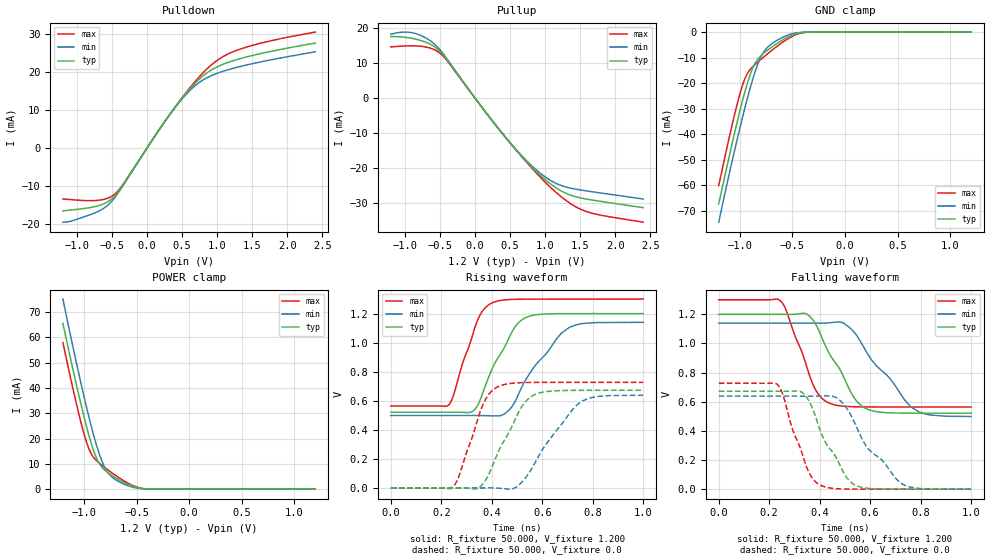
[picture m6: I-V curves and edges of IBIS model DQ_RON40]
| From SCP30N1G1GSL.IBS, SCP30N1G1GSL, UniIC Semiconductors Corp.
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|   Model DQ_RON40
[Model] DQ_RON40
Model_type I/O
Vinl =  0.500V
Vinh =  0.700V
Vmeas =  0.600V
Rref =  50.000
Vref =  0.600V
C_comp   1.373pF   1.353pF   1.403pF
[Model Spec]
Vinh   0.700V   0.670V   0.750V
Vinl   0.500V   0.470V   0.550V
Vmeas   0.600V   0.570V   0.650V
Vref   0.600V   0.570V   0.650V
Rref   50.000   NA   NA
[Temperature Range]   25.000   85.000   -40.000
[Voltage Range]   1.200V   1.140V   1.300V
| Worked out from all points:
|   slope of the pulldown table from 0 to 0.18 V, typ, clamps not added: 36 ohm
|   slope of the pullup table from 0 to 0.18 V, typ, clamps not added: 37.6 ohm
|   GND clamp passes 1 mA (typ) near -0.49 V on its own axis
|   POWER clamp passes 1 mA (typ) near -0.53 V on its own axis
|   rising waveform, R_fixture 50.000, V_fixture 1.200: 20-80 % time 112ps typ, 150ps min, 82.8ps max; typ from 0.522 V to 1.2 V
|   rising waveform, R_fixture 50.000, V_fixture 0.0: 20-80 % time 113ps typ, 151ps min, 85ps max; typ from 0 V to 0.672 V
|   falling waveform, R_fixture 50.000, V_fixture 1.200: 20-80 % time 124ps typ, 169ps min, 93ps max; typ from 1.2 V to 0.522 V
|   falling waveform, R_fixture 50.000, V_fixture 0.0: 20-80 % time 113ps typ, 155ps min, 84.2ps max; typ from 0.672 V to 0 V
[Pulldown]
|Voltage   I(typ)   I(min)   I(max)
-1.2V     -16.5mA    -19.45mA   -13.36mA
-719mV    -15.25mA   -16.82mA   -13.74mA
-571mV    -14.22mA   -15.18mA   -13.24mA
-460mV    -12.61mA   -13.01mA   -12.11mA
-349mV    -9.901mA   -10.03mA   -9.712mA
317mV     8.617mA    8.575mA    8.603mA
576mV     14.77mA    14.41mA    14.99mA
761mV     18.31mA    17.39mA    18.99mA
1.02V     21.44mA    19.72mA    23.23mA
1.279V    23.17mA    21.14mA    25.61mA
1.723V    25.17mA    22.96mA    27.94mA
2.4V      27.51mA    25.23mA    30.4mA
[Pullup]
|Voltage   I(typ)   I(min)   I(max)
-1.2V     17.52mA    18.2mA     14.6mA
-1.004V   17.34mA    18.82mA    14.85mA
-819mV    16.67mA    18.22mA    14.85mA
-634mV    15.31mA    16.3mA     14.22mA
-486mV    13.07mA    13.48mA    12.58mA
69mV      -1.852mA   -1.865mA   -1.826mA
439mV     -11.32mA   -11.29mA   -11.28mA
772mV     -18.89mA   -18.59mA   -19.14mA
1.031V    -23.77mA   -22.92mA   -24.59mA
1.29V     -27.13mA   -25.36mA   -29.11mA
1.549V    -28.68mA   -26.39mA   -32.09mA
2.4V      -31.3mA    -28.83mA   -35.44mA
[GND_clamp]
|Voltage   I(typ)   I(min)   I(max)
-1.2V     -67.26mA   -74.42mA   -60.1mA
-1.05V    -39.62mA   -46.47mA   -32.4mA
-1V       -31.05mA   -37.77mA   -24.37mA
-950mV    -23.16mA   -29.46mA   -18.1mA
-925mV    -19.62mA   -25.5mA    -16.02mA
-875mV    -13.89mA   -18.21mA   -13.48mA
-825mV    -10.4mA    -12.16mA   -11.61mA
-775mV    -8.365mA   -7.964mA   -9.852mA
-700mV    -6.001mA   -4.671mA   -7.319mA
-525mV    -1.587mA   -933.3uA   -2.208mA
-375mV    -90.13uA   -49.22uA   -132.9uA
1.2V      0A         0A         0A
[POWER_clamp]
|Voltage   I(typ)   I(min)   I(max)
-1.2V     65.51mA    75.11mA    57.91mA
-1.05V    37.38mA    45.87mA    29.99mA
-1V       28.74mA    36.73mA    21.95mA
-950mV    20.85mA    28.08mA    15.65mA
-925mV    17.34mA    24.01mA    13.56mA
-875mV    11.74mA    16.61mA    11.06mA
-825mV    8.457mA    10.65mA    9.317mA
-775mV    6.603mA    6.7mA      7.708mA
-725mV    5.177mA    4.492mA    6.178mA
-550mV    1.336mA    943.1uA    1.707mA
-400mV    85.95uA    67.55uA    91.19uA
1.2V      0A         0A         0A
[Ramp]
| variable   typ   min   max
dV/dt_r   0.403/0.113n   0.383/0.151n   0.436/85.122p
dV/dt_f   0.407/0.123n   0.385/0.168n   0.441/93.034p
R_load = 50.000
[Rising Waveform]
R_fixture= 50.000
V_fixture= 1.200
V_fixture_min= 1.140
V_fixture_max= 1.300
|time   V(typ)   V(min)   V(max)
0s        521.6mV    498.6mV    564.2mV
229ps     521.7mV    498.6mV    570.4mV
331ps     537.9mV    498.8mV    1.093V
363ps     648.1mV    498.2mV    1.217V
404ps     830mV      496mV      1.276V
472ps     1.046V     543.4mV    1.297V
522ps     1.161V     704.9mV    1.299V
658ps     1.199V     1.029V     1.3V
708ps     1.2V       1.106V     1.3V
1ns       1.2V       1.14V      1.3V
[Rising Waveform]
R_fixture= 50.000
V_fixture= 0.0
V_fixture_min= 0.0
V_fixture_max= 0.0
|time   V(typ)   V(min)   V(max)
0s        38.4nV     122.4nV    22.61nV
246ps     132.9uV    -10.17uV   8.174mV
270ps     387.1uV    -19.6uV    81.65mV
354ps     8.179mV    234.7uV    523.9mV
391ps     103.8mV    526.7uV    650.6mV
430ps     265.3mV    -1.714mV   700.7mV
503ps     509.9mV    13.72mV    723.6mV
572ps     643.8mV    175.8mV    726.5mV
759ps     672mV      598.2mV    726.9mV
1ns       672.2mV    638.4mV    726.9mV
[Falling Waveform]
R_fixture= 50.000
V_fixture= 1.200
V_fixture_min= 1.140
V_fixture_max= 1.300
|time   V(typ)   V(min)   V(max)
0s        1.2V       1.14V      1.3V
243ps     1.2V       1.14V      1.295V
265ps     1.2V       1.14V      1.237V
354ps     1.196V     1.14V      810.6mV
393ps     1.104V     1.14V      655.7mV
433ps     947mV      1.141V     594.7mV
512ps     705.3mV    1.118V     567.5mV
592ps     546.7mV    922.9mV    564.5mV
793ps     521.7mV    530.6mV    564.2mV
1ns       521.6mV    498.8mV    564.2mV
[Falling Waveform]
R_fixture= 50.000
V_fixture= 0.0
V_fixture_min= 0.0
V_fixture_max= 0.0
|time   V(typ)   V(min)   V(max)
0s        672.2mV    638.4mV    726.9mV
235ps     672.1mV    638.4mV    714.1mV
340ps     649.7mV    638.3mV    192.4mV
369ps     565.6mV    638.4mV    80.17mV
412ps     359.1mV    639.3mV    20.39mV
476ps     180mV      616.5mV    2.572mV
530ps     39.12mV    486.5mV    446.4uV
585ps     6.991mV    293.1mV    74.09uV
726ps     77.88uV    36.72mV    755nV
1ns       48.27nV    10.39uV    18.02nV
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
